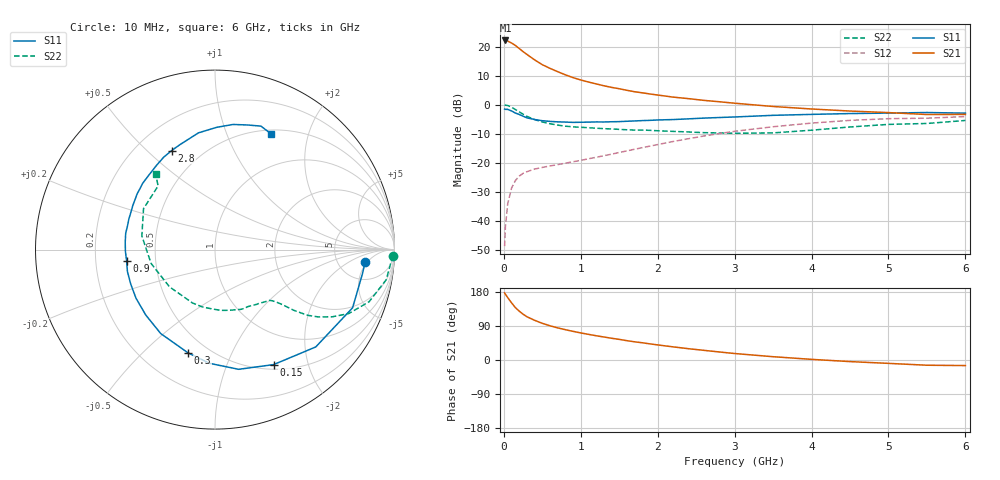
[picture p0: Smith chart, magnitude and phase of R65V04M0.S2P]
! SIEMENS Small Signal Semiconductors
! BFR193
! Si NPN RF Bipolar Junction Transistor in SOT23
! VCE = 5 V  IC = 4 mA
! Common Emitter S-Parameters:  May  1996
# GHz  S  MA  R  50
!  f  S11  S21  S12  S22
! GHz  MAG  ANG  MAG  ANG  MAG  ANG  MAG  ANG
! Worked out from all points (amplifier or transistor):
!   36 points, 10 MHz to 6 GHz, reference 50 ohm
!   highest |S21| = 22.1 dB at 20 MHz (marker M1)
!   |S21| within 3 dB of that: start of sweep to 210.4 MHz
!   unconditionally stable (mu >= 1): 963.5 MHz to 1.978 GHz
!   at 250 MHz: K = 0.37, MSG = 20.9 dB, |S12| = -23.6 dB
!   at 1.4 GHz: K = 1.07, MAG = 9.8 dB, |S12| = -17.0 dB
!   at 6 GHz: K = 0.97, MSG = 0.4 dB, |S12| = -4.1 dB
!   S11 on the Smith chart (normalised r, x): 10 MHz: 9, -4; 150 MHz: 0.56, -1.48; 300 MHz: 0.39, -0.70; 900 MHz: 0.34, -0.06; 2.8 GHz: 0.35, +0.60; 6 GHz: 0.55, +1.45
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0.01  0.8398 -4.7  12.6 177.1  0.0037 84.0  0.9935 -2.0
0.02  0.8323 -9.4  12.72 173.6  0.0079 87.1  0.9832 -4.1
0.05  0.8324 -22.9  12.42 164.8  0.0197 79.5  0.9686 -10.0
0.1  0.7806 -44.0  11.5 151.0  0.0369 68.3  0.9063 -18.7
0.15  0.7191 -63.0  10.44 138.2  0.0496 60.3  0.8255 -25.6
0.2  0.6799 -78.8  9.236 128.9  0.0591 54.7  0.7532 -29.8
0.25  0.6345 -92.7  8.18 120.8  0.0661 50.1  0.6872 -33.1
0.3  0.5947 -104.6  7.315 114.2  0.0705 47.6  0.6311 -35.4
0.4  0.557 -122.9  5.9 104.7  0.0783 44.9  0.5544 -37.6
0.5  0.5306 -136.7  4.875 96.8  0.0836 44.2  0.505 -38.7
0.6  0.5168 -148.4  4.217 90.3  0.0885 44.7  0.4709 -39.7
0.7  0.5073 -157.8  3.695 84.7  0.0935 46.2  0.4459 -40.7
0.9  0.4966 -172.6  2.92 75.6  0.1048 49.3  0.416 -42.9
1.1  0.5019 175.2  2.454 67.7  0.1177 52.6  0.4018 -46.5
1.3  0.505 165.0  2.118 60.7  0.133 55.6  0.3876 -50.3
1.6  0.5194 151.9  1.768 51.0  0.1607 58.5  0.3706 -57.8
2.2  0.5555 131.3  1.351 34.7  0.2331 58.8  0.3477 -76.6
2.8  0.6024 113.6  1.124 21.2  0.3186 53.5  0.3271 -102.6
3.5  0.6568 98.1  0.932 8.7  0.4181 42.5  0.3276 -140.8
4.5  0.7044 81.8  0.778 -4.2  0.5379 25.1  0.4146 169.4
5.5  0.7341 69.6  0.678 -13.8  0.5868 7.1  0.4757 131.8
6  0.7163 64.1  0.681 -14.7  0.6249 2.0  0.5359 128.1
